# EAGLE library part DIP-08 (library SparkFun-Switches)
8-Position DIP Switch 8-circuit DIP (dual inline package) switch. Commonly used to physcially set a circuit's behavior. SparkFun Products DIP Switch - 8 Position (COM-08034)
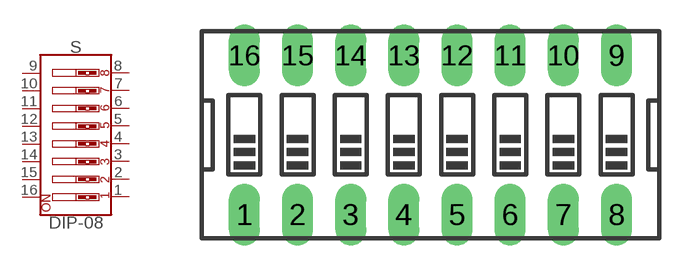
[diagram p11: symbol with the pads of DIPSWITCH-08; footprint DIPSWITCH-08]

Designator prefix S

## DIP-08-PTH (PROD_ID: SWCH-12197; SF_SKU: COM-08034)  [DIPSWITCH-08]
1  1  pas
2  2  pas
3  3  pas
4  4  pas
5  5  pas
6  6  pas
7  7  pas
8  8  pas
9  9  pas
10  10  pas
11  11  pas
12  12  pas
13  13  pas
14  14  pas
15  15  pas
16  16  pas

## Footprint DIPSWITCH-08 (pad centres in mm)
8-Position DIP Switch - PTH, 0.1"-Pitch Standard size through-hole DIP switch, 2.54 mm / 0.1" pitch Datasheet
drill 0.97 long: 1 -8.89,-3.81; 2 -6.35,-3.81; 3 -3.81,-3.81; 4 -1.27,-3.81; 5 1.27,-3.81; 6 3.81,-3.81; 7 6.35,-3.81; 8 8.89,-3.81; 9 8.89,3.81; 10 6.35,3.81; 11 3.81,3.81; 12 1.27,3.81; 13 -1.27,3.81; 14 -3.81,3.81; 15 -6.35,3.81; 16 -8.89,3.81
